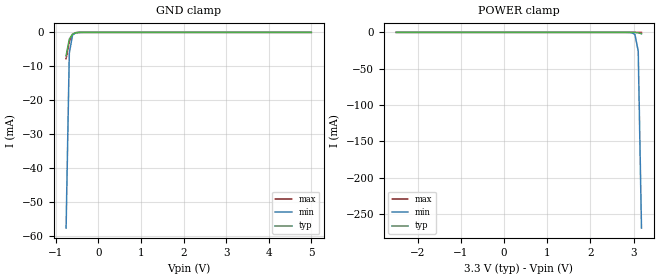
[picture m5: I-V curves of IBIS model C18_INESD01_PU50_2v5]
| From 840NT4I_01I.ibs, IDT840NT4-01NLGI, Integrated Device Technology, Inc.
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| 3.25758e+00   -6.92224e-03   -1.23527e+00   -1.07149e-03
| 3.33333e+00   -4.29506e-02   -2.23637e+00   -4.11997e-03
| 3.40909e+00   -5.86135e-01   -3.23815e+00   -1.02974e-02
| 3.48485e+00   -1.79017e+00   -4.24043e+00   -2.01278e-02
| 3.56061e+00   -2.99495e+00   -5.24309e+00   -7.87092e-02
| 3.63636e+00   -4.20024e+00   -6.24602e+00   -1.11369e+00
| 3.71212e+00   -5.40590e+00   -7.24916e+00   -2.65555e+00
| 3.78788e+00   -6.61182e+00   -8.25246e+00   -4.19783e+00
| 3.86364e+00   -7.81792e+00   -9.25587e+00   -5.74035e+00
| 3.93939e+00   -9.02412e+00   -1.02594e+01   -7.28299e+00
| 4.01515e+00   -1.02304e+01   -1.12629e+01   -8.82567e+00
| 4.09091e+00   -1.14366e+01   -1.22664e+01   -1.03683e+01
| 4.16667e+00   -1.26429e+01   -1.32700e+01   -1.19109e+01
| 4.24242e+00   -1.38491e+01   -1.42735e+01   -1.34534e+01
| 4.31818e+00   -1.50552e+01   -1.52769e+01   -1.49957e+01
| 4.39394e+00   -1.62613e+01   -1.62803e+01   -1.65379e+01
| 4.46970e+00   -1.74672e+01   -1.72837e+01   -1.80799e+01
| 4.54545e+00   -1.86730e+01   -1.82870e+01   -1.96217e+01
| 4.62121e+00   -1.98787e+01   -1.92902e+01   -2.11633e+01
| 4.69697e+00   -2.10843e+01   -2.02933e+01   -2.27047e+01
| 4.77273e+00   -2.22897e+01   -2.12963e+01   -2.42459e+01
| 4.84848e+00   -2.34950e+01   -2.22993e+01   -2.57868e+01
| 4.92424e+00   -2.47001e+01   -2.33021e+01   -2.73276e+01
| 5.00000e+00   -2.59051e+01   -2.43049e+01   -2.88681e+01
[Model] C18_INESD01_PU50_2v5
Model_type   Input
Polarity   Non-Inverting
Vinl = 0.8V
Vinh = 2.0V
|   typ   min   max
C_comp   2pF   1.5pF   2.5pF
|   typ   min   max
[Voltage range]   3.3V   3.135V   3.465V
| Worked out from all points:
|   GND clamp passes 1 mA (typ) near -0.63 V on its own axis
[GND_clamp]
|Voltage   I (typ)   I (min)   I (max)
|Note, modeling breaks down at 250mA and above.  This is well beyond the functional   |
|operating range of the device.  Should this scenario occur, catastrophic failure and   |
|possible damage to the device and/or board is of higher concern than the I-V curve   |
|behavior.  The IBIS checker will flag currents in excess of 10A with warnings.  Lines   |
|with currents in excess of 0.35 A have been commented out.  The points still remain|
|available to the user if the user desires to use them.   |
|-2.50000e+00   -2.59051e+01   -2.26503e+01   -3.14095e+01
|-2.42424e+00   -2.47001e+01   -2.16474e+01   -2.98694e+01
|-2.34848e+00   -2.34949e+01   -2.06444e+01   -2.83289e+01
|-2.27273e+00   -2.22897e+01   -1.96413e+01   -2.67883e+01
|-2.19697e+00   -2.10842e+01   -1.86381e+01   -2.52475e+01
|-2.12121e+00   -1.98787e+01   -1.76349e+01   -2.37064e+01
|-2.04545e+00   -1.86730e+01   -1.66315e+01   -2.21652e+01
|-1.96970e+00   -1.74672e+01   -1.56281e+01   -2.06237e+01
|-1.89394e+00   -1.62612e+01   -1.46247e+01   -1.90820e+01
|-1.81818e+00   -1.50552e+01   -1.36212e+01   -1.75402e+01
|-1.74242e+00   -1.38491e+01   -1.26176e+01   -1.59981e+01
|-1.66667e+00   -1.26429e+01   -1.16141e+01   -1.44559e+01
|-1.59091e+00   -1.14366e+01   -1.06106e+01   -1.29135e+01
|-1.51515e+00   -1.02304e+01   -9.60708e+00   -1.13710e+01
|-1.43939e+00   -9.02411e+00   -8.60364e+00   -9.82839e+00
|-1.36364e+00   -7.81791e+00   -7.60030e+00   -8.28572e+00
|-1.28788e+00   -6.61181e+00   -6.59709e+00   -6.74304e+00
|-1.21212e+00   -5.40589e+00   -5.59408e+00   -5.20043e+00
|-1.13636e+00   -4.20023e+00   -4.59132e+00   -3.65798e+00
|-1.06061e+00   -2.99494e+00   -3.58889e+00   -2.11583e+00
|-9.84848e-01   -1.79016e+00   -2.58692e+00   -5.74171e-01
|-9.09091e-01   -5.86126e-01   -1.58556e+00   -3.88817e-02
|-8.33333e-01   -4.29412e-02   -5.85042e-01   -1.59892e-02
-757.6mV  -6.913mA   -57.82mA   -7.776mA
-681.8mV  -2.01mA    -6.108mA   -2.699mA
-606.1mV  -502.7uA   -806.7uA   -594.1uA
-530.3mV  -96.99uA   -129.6uA   -89.62uA
-378.8mV  -2.15uA    -5.029uA   -802.4nA
5V        190.2pA    660.4pA    165.4pA
[Power_clamp]
|Voltage   I (typ)   I (min)   I (max)
|Note, modeling breaks down at 250mA and above.  This is well beyond the functional   |
|operating range of the device.  Should this scenario occur, catastrophic failure and   |
|possible damage to the device and/or board is of higher concern than the I-V curve   |
|behavior.  The IBIS checker will flag currents in excess of 10A with warnings.  Lines   |
|with currents in excess of 0.35 A have been commented out.  The points still remain|
|available to the user if the user desires to use them.   |
-2.5V     190.2pA    642.1pA    169.5pA
2.803V    -276.8nA   -13.47uA   -287.7pA
2.955V    -15.35uA   -417.6uA   -144.4nA
3.03V     -96.99uA   -2.929mA   -1.924uA
3.106V    -502.7uA   -25.77mA   -21.68uA
3.182V    -2.01mA    -269.5mA   -180.4uA
